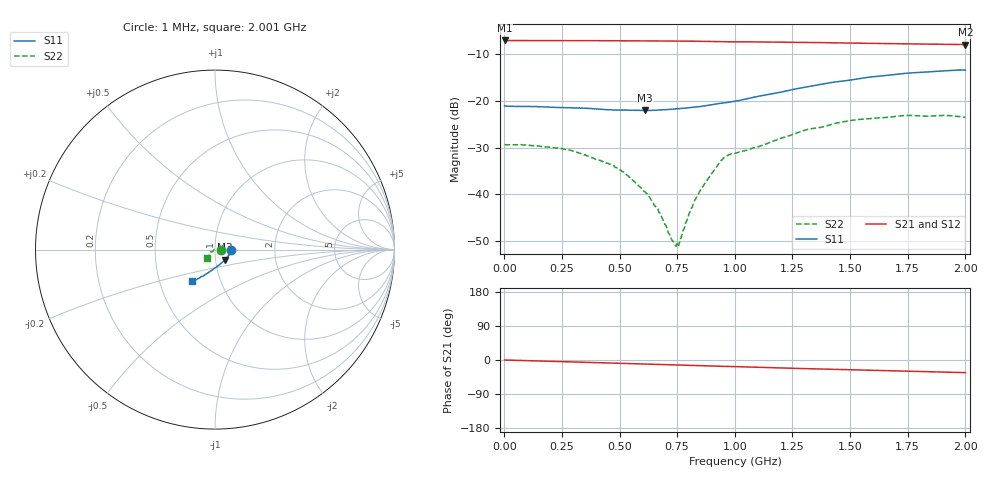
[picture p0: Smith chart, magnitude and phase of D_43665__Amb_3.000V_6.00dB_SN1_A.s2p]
! device id: 43665_
! dir: \\malibu\benchdata\1_engineers\tn_data\43665_75ohm\new\sparar\43665_\amb\3p000v\6p00db
! Serial: 1
! Insertion: A
! Temp: Amb
! VDD: 3.000V
! Attenuation Step: 6.00dB
! IDD: 1.455118e+00mA
! FILE NAME
! DATE 03-27-2009 08:34:50
! CORRECTED  DATA
#  Hz  S  RI  R  75
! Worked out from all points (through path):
!   401 points, 1 MHz to 2.001 GHz, reference 75 ohm
!   highest |S21| = -7.05 dB at 1 MHz (marker M1); lowest = -7.9 dB at 2.001 GHz (marker M2)
!   group delay of S21, straight-line fit = 47.2 ps
!   lowest |S11| = -22.1 dB at 611 MHz (marker M3), VSWR 1.17, Z = 83.2 - j9.42 ohm
!   |S11| at or under -10 dB: start of sweep to end of sweep
!   |S22| runs from -51.1 to -23.1 dB; largest |S21 - S12| = 0.0016
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1000000  0.0884 -0.000957  0.4439 -0.000718  0.4439 -0.00059  0.0343 -0.000326
2.41e8  0.0823 -0.0208  0.4414 -0.0319  0.4415 -0.032  0.0299 0.00803
3.36e8  0.0785 -0.0294  0.4397 -0.0446  0.4399 -0.0447  0.025 0.0106
4.56e8  0.0695 -0.04  0.4369 -0.0605  0.437 -0.0607  0.0185 0.00998
4.96e8  0.0662 -0.0445  0.4357 -0.0659  0.4358 -0.0661  0.0159 0.00993
5.26e8  0.0639 -0.0475  0.4346 -0.0699  0.4347 -0.07  0.0137 0.00942
6.11e8  0.0553 -0.0562  0.4314 -0.0808  0.4314 -0.081  0.00731 0.00769
6.71e8  0.0492 -0.063  0.4292 -0.0888  0.4292 -0.0888  0.00357 0.00525
7.36e8  0.0416 -0.0703  0.4263 -0.0975  0.4264 -0.0974  -0.000563 0.00299
7.51e8  0.04 -0.072  0.4256 -0.0995  0.4256 -0.0994  -0.0018 0.00247
7.66e8  0.0381 -0.0737  0.4248 -0.1015  0.4248 -0.1015  -0.00304 0.00152
8.16e8  0.0317 -0.0792  0.4221 -0.1082  0.422 -0.1082  -0.00696 -0.00225
8.56e8  0.0256 -0.0835  0.4196 -0.1136  0.4195 -0.1135  -0.00989 -0.00621
9.41e8  0.0129 -0.0934  0.4124 -0.1235  0.4126 -0.1233  -0.0192 -0.0128
9.71e8  0.00921 -0.0962  0.4108 -0.1257  0.411 -0.1255  -0.0233 -0.012
1.001e9  0.00475 -0.0991  0.4097 -0.1286  0.4099 -0.1285  -0.0245 -0.0122
1.336e9  -0.0485 -0.1358  0.3873 -0.1666  0.3878 -0.1668  -0.035 -0.0365
1.506e9  -0.0746 -0.1503  0.3735 -0.1829  0.3739 -0.1834  -0.04 -0.047
1.671e9  -0.0965 -0.1623  0.3605 -0.197  0.3602 -0.1977  -0.0424 -0.0519
1.746e9  -0.1055 -0.1672  0.3544 -0.2028  0.3544 -0.2038  -0.0435 -0.0545
1.911e9  -0.1207 -0.1721  0.3419 -0.2143  0.3415 -0.2144  -0.0459 -0.0527
2.001e9  -0.1264 -0.1727  0.3353 -0.2202  0.3339 -0.2211  -0.0444 -0.0494
